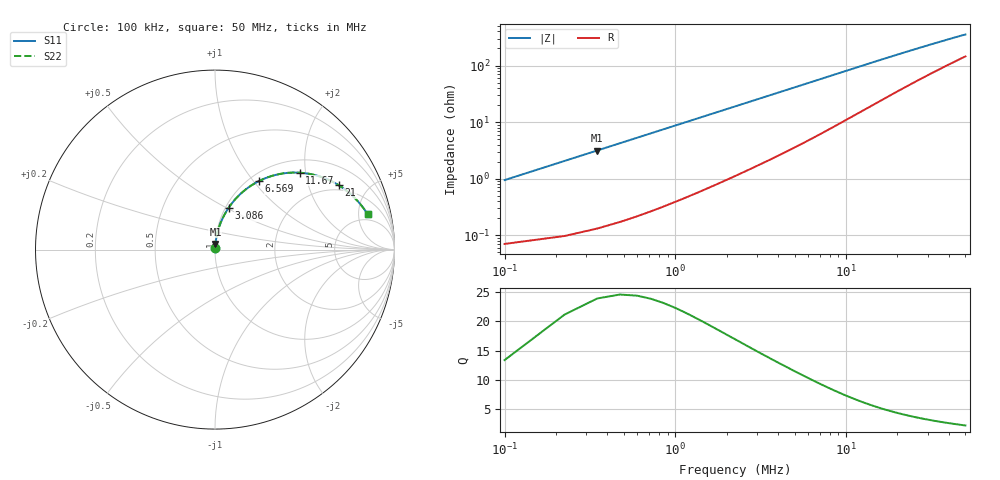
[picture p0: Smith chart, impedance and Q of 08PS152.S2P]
! Coilcraft 0805PS-152 Power Chip Inductor
! 5 February 2003
# MHZ S MA R 50
!Freq  MagS11  AngS11  MagS21  AngS21  MagS12  AngS12  MagS22  AngS22
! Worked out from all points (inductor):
!   403 points, 100 kHz to 50 MHz, reference 50 ohm
!   read as one part in series: L = 1.42 uH near 348.8 kHz
!   highest Q = 23.2 at 348.8 kHz (marker M1), where L = 1.43 uH
!   S11 on the Smith chart (normalised r, x): 100 kHz: 1.00, +0.02; 3.086 MHz: 1.03, +0.51; 6.569 MHz: 1.11, +1.07; 11.67 MHz: 1.28, +1.85; 21 MHz: 1.76, +3.18; 50 MHz: 3.90, +6.45
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0.1  0.009433 85.2  0.9993 -0.5  0.9993 -0.5  0.009433 85.2
0.2244  0.02054 86.1  0.9988 -1.2  0.9988 -1.2  0.02054 86.1
0.3488  0.03141 85.8  0.9982 -1.8  0.9982 -1.8  0.03141 85.8
0.4732  0.04212 85.3  0.9974 -2.4  0.9974 -2.4  0.04212 85.3
0.5976  0.0527 84.6  0.9965 -3.0  0.9965 -3.0  0.0527 84.6
0.722  0.06316 84.0  0.9954 -3.6  0.9954 -3.6  0.06316 84.0
0.9708  0.0838 82.6  0.9928 -4.8  0.9928 -4.8  0.0838 82.6
1.2196  0.1041 81.3  0.9897 -6.0  0.9897 -6.0  0.1041 81.3
1.5928  0.1339 79.4  0.9841 -7.7  0.9841 -7.7  0.1339 79.4
1.966  0.1629 77.4  0.9776 -9.4  0.9776 -9.4  0.1629 77.4
2.4636  0.2004 74.9  0.9675 -11.5  0.9675 -11.5  0.2004 74.9
3.0856  0.2454 71.9  0.9529 -14.2  0.9529 -14.2  0.2454 71.9
4.5784  0.3438 65.2  0.9111 -20.0  0.9111 -20.0  0.3438 65.2
6.5688  0.4535 57.3  0.8462 -26.8  0.8462 -26.8  0.4535 57.3
8.4348  0.5351 51.0  0.783 -32.1  0.783 -32.1  0.5351 51.0
11.6692  0.637 42.3  0.6806 -39.0  0.6806 -39.0  0.637 42.3
16.7696  0.7315 32.8  0.5528 -45.8  0.5528 -45.8  0.7315 32.8
20.9992  0.7767 27.5  0.4753 -49.1  0.4753 -49.1  0.7767 27.5
25.1044  0.8055 23.8  0.418 -51.0  0.418 -51.0  0.8055 23.8
33.4392  0.8407 18.6  0.3367 -52.9  0.3367 -52.9  0.8407 18.6
41.774  0.8606 15.3  0.2836 -53.2  0.2836 -53.2  0.8606 15.3
50  0.8732 13.0  0.2469 -52.8  0.2469 -52.8  0.8732 13.0
